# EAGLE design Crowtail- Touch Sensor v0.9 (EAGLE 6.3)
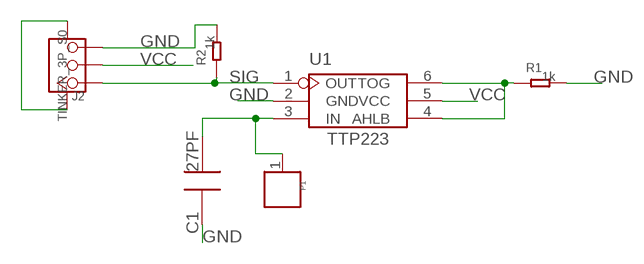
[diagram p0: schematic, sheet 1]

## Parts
C1  27PF  C0603  [0603]
J2  TINKER_3P_S0  [TINKER_3P_S0]
P1  PAD'D450MIL'  [1P-D450]
R1  1k  R0603  [0603]
R2  1k  R0603  [0603]
U1  TTP223  [SOT23-6L]

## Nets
GND: C1.1 J2.3 J2.SS1 J2.SS2 R1.2 R2.2 U1.2(GND)
IN: C1.2 P1.1 U1.3(IN)
N$2: R1.1 U1.4(AHLB) U1.6(TOG)
SIG: J2.1 R2.1 U1.1(OUT)
VCC: J2.2 U1.5(VCC)

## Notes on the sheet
- TTP223

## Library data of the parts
C1 = CPT_SMD:C0603; C0603: 100N
J2 = Connector:TINKER_3P_S0
P1 = Discrete:PAD
R1 R2 = CPT_SMD:R0603
U1 = Seeed:TTP223

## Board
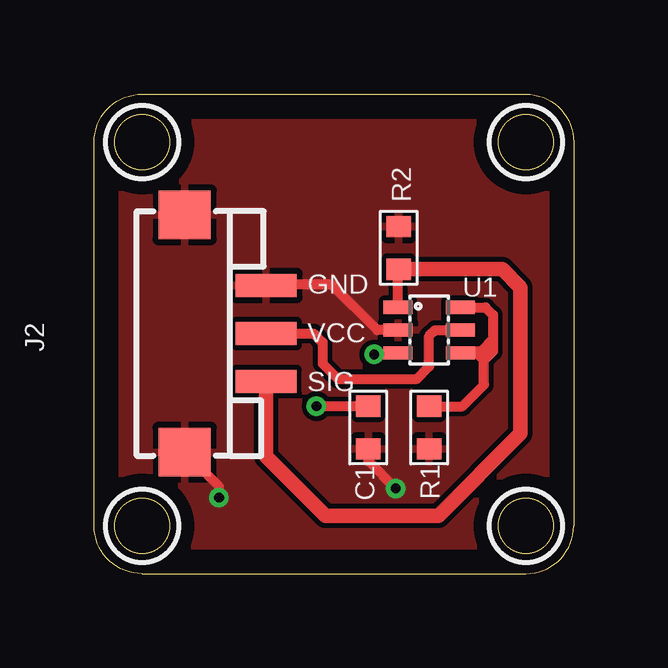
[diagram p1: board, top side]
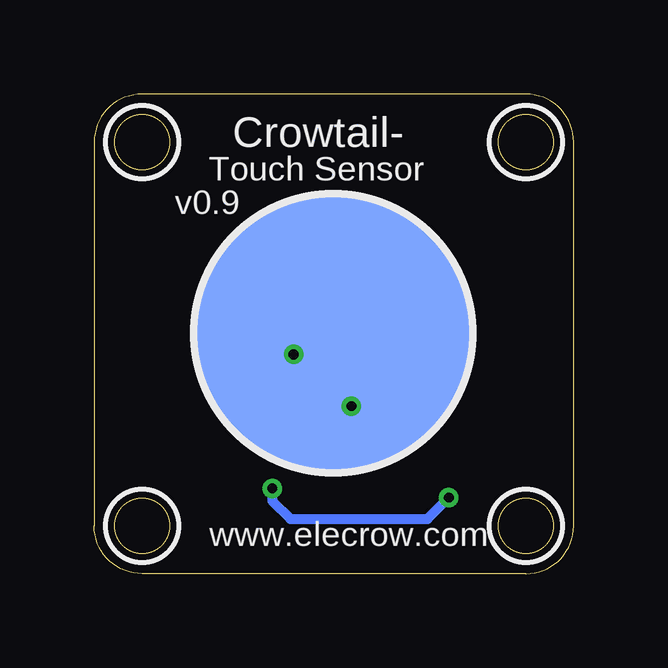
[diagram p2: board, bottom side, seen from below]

Size 20 x 20 mm. Coordinates in mm from the lower left corner, seen from the top.
Outline: 2,0 18,0 arc90 20,2 20,18 arc90 18,20 2,20 arc90 0,18 0,2 arc90 2,0
Outline: circle at 2,18 radius 1.14
Outline: circle at 18,18 radius 1.14
Outline: circle at 2,2 radius 1.14
Outline: circle at 18,2 radius 1.14
Copper layers (1*16): Top 0.035mm / dielectric 1.5mm / Bottom 0.035mm
Design rules "default *": minimum track width 10mil, minimum drill 24mil, track to track 8mil, track to pad 8mil, pad to pad 8mil, via to via 8mil, smd to smd 8mil, copper to edge 40mil, drill to drill 8mil, minimum pad ring 10mil, minimum via ring 8mil, stop-mask expansion 2mil, vias tented up to drill 100mil, thermal gap 10mil
tRestrict: area 0.5,16.5 to 3.5,19.5; area 16.5,16.5 to 19.5,19.5; area 0.5,0.5 to 3.5,3.5; area 16.5,0.5 to 19.5,3.5
bRestrict: area 0.5,16.5 to 3.5,19.5; area 16.5,16.5 to 19.5,19.5; area 0.5,0.5 to 3.5,3.5; area 16.5,0.5 to 19.5,3.5

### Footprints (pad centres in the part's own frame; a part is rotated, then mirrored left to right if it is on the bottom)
0603 = smd 0.889 x 1.016: 1 -0.889,0; 2 0.889,0
TINKER_3P_S0 = smd 0.965 x 2.54: 1 -1.984,-3.175; 2 0.016,-3.175; 3 2.016,-3.175 | smd 2.032 x 2.184: SS1 -4.93,0.225; SS2 4.962,0.225
1P-D450 = smd 11.43 x 11.43: 1 0,0
SOT23-6L = smd 0.55 x 1.2: 1 -0.95,-1.3; 2 0,-1.3; 3 0.95,-1.3; 4 0.95,1.3; 5 0,1.3; 6 -0.95,1.3

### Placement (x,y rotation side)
C1  11.43,6.1 90 top
J2  4,10 90 top
P1  10,10 0 bottom
R1  13.97,6.1 270 top
R2  12.7,13.59 90 top
U1  13.97,10.16 270 top

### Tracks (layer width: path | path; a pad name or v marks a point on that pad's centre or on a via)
GND  (via drill 0.41)
  Top 0.406: U1.2 11.81,10.16 9.91,12.06 7.22,12.06 J2.3 | C1.1 11.43,4.7 v12.57,3.56 | v5.21,3.17 5.21,3.64 J2.SS1
  Bottom 0.406: v12.57,3.56 12.57,3.05 11.81,2.29 6.1,2.29 v5.21,3.17
  pour Top: 0,0 20.32,0 20.32,20.32 0,20.32
IN  (via drill 0.41)
  Top 0.406: v11.68,9.14 12.6,9.14 U1.3 | C1.2 v9.27,6.99
  Bottom 0.406: v11.68,9.14 11.3,9.14 10.45,10 P1.1 9.27,9.27 v9.27,6.99
N$2
  Top 0.406: 16.64,9.27 16.38,9.27 | 16.38,9.27 16.13,9.27 | 16.13,9.27 15.88,9.27 | 15.88,9.27 15.33,9.27 U1.4 | 16.26,8.89 16.26,7.87 15.37,6.99 R1.1 | 16.26,8.89 16.26,9.14 16.38,9.27 | 16.26,8.89 16.64,9.27 | 16.26,8.89 15.88,9.27 | U1.6 16.32,11.11 16.64,10.79 16.64,9.78 | 16.64,9.78 16.64,9.27 | 16.64,9.78 16.13,9.27
SIG
  Top 0.406: U1.1 12.67,12.67 R2.1
  Top 0.61: J2.1 7.17,4.89 9.65,2.41 14.35,2.41 17.78,5.84 17.78,11.94 17.02,12.7 R2.1
VCC
  Top 0.406: U1.5 14.22,10.16 13.97,9.91 13.97,8.64 13.46,8.13 10.16,8.13 9.53,8.76 9.53,9.65 9.16,10.02 J2.2

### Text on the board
tPlace: GND | VCC | SIG
bPlace: Crowtail- | Touch Sensor | v0.9 | www.elecrow.com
